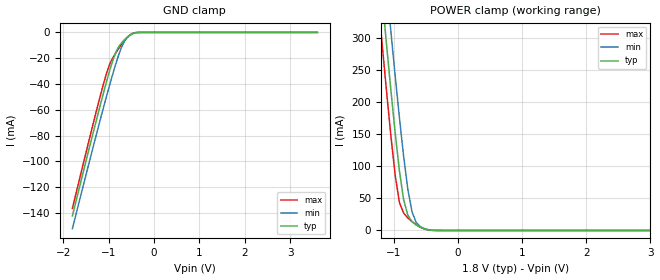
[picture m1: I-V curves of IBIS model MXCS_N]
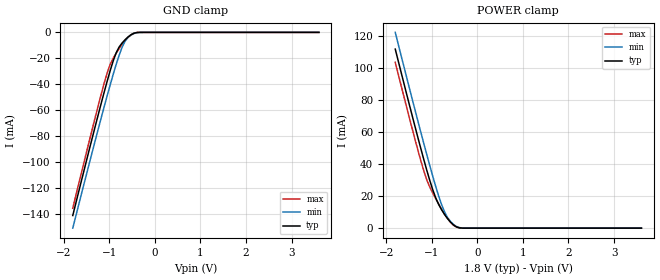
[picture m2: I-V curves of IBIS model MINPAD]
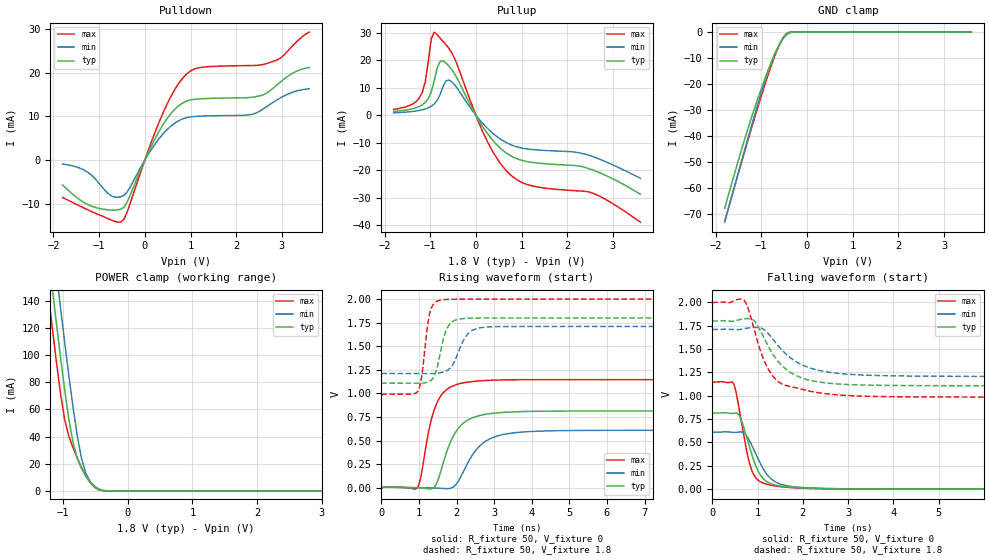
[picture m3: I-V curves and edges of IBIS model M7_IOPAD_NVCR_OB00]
| Created by SiliconSmart  O-2018.09-SP2-3
[IBIS Ver]   4.0
[File Name]   as10204wa_rev1p4.ibs
[File Rev]   1.4
[Date]   Thursday Mar 21 2024
|[Source]   Avalanche Team
|[Notes]   Generated IBIS models from Silicon Smart
|[Rev 1.0]  Initial Release based on extracted netlist
|   Characterization
|[Rev 1.1]  Update Package RLC
|[Rev 1.2]  Recharacterize MIOPAD with Hspice run in high accuracy mode
|[Rev 1.3]  Recharacterize with Hspice to align with datasheet parameter
|[Rev 1.4]  Update the pin to the package pinout assignment
|[Disclaimer]   THE MODEL LIBRARIES ARE PROVIDED AS IS.
|[Copyright]   Copyright 2019, Avalanche Technology., All Rights Reserved
[Component]   AS10xx204_WSON
[Manufacturer] Avalanche Technology
| CONTENT :
| This file contains IBIS MODEL for PSRAM device
| AS1001204 AS1004204 AS1008204 AS1016204
| USAGE :
| The models are derived for the 1.71V to 2.0V I/O Operation.
| Temperatures for model generation: typ: 25, max: -40, min: 105
| Voltages : typ: 1.8V, min: 1.71V, max: 2.0V
| PACKAGES SUPPORTED :
| 8-pad WSON (5.0mm x 6.0mm)
| VERIFICATION :
| Errors  : 0
| Warnings: 30
| All warnings due to non-monotonic data
[Package]
|variable   typ   min   max
R_pkg   8.90E-04   8.89E-04  8.91E-04
L_pkg   1.185E-09  1.18E-09  1.19E-09
C_pkg   2.30E-13   2.21E-13  2.39E-13
[Pin]   signal_name   model_name   R_pin   L_pin   C_pin
1   CS#   MXCS_N   1.05E-01  1.35E-09  9.16E-14
2   SO   MIOPAD   1.05E-01  1.35E-09  9.16E-14
3   WP#   MIOPAD   1.05E-01  1.35E-09  9.16E-14
5   SI   MIOPAD   3.75E-02  3.89E-10  4.24E-14
6   CLK   MINPAD   3.75E-02  3.89E-10  4.24E-14
7   IO_3   MIOPAD   3.75E-02  3.89E-10  4.24E-14
4   VSS   GND   NA   NA   NA
8   VCC   POWER   NA   NA   NA
[Model Selector] MIOPAD
| Model Description
M0_IOPAD_NVCR_OB07   20 Ohms drv strength
M1_IOPAD_NVCR_OB06   30 Ohms drv strength
M2_IOPAD_NVCR_OB05   60 Ohms drv strength
M3_IOPAD_NVCR_OB04   45 Ohms drv strength
M4_IOPAD_NVCR_OB03   70 Ohms drv strength
M5_IOPAD_NVCR_OB02   90 Ohms drv strength
M6_IOPAD_NVCR_OB01   120 Ohms drv strength
M7_IOPAD_NVCR_OB00   45 Ohms drv strength
| Models and submodels in the file (10): MXCS_N (Input), MINPAD (Input), M7_IOPAD_NVCR_OB00 (I/O), M3_IOPAD_NVCR_OB04 (I/O), M5_IOPAD_NVCR_OB02 (I/O), M1_IOPAD_NVCR_OB06 (I/O), M6_IOPAD_NVCR_OB01 (I/O), M2_IOPAD_NVCR_OB05 (I/O), M4_IOPAD_NVCR_OB03 (I/O), M0_IOPAD_NVCR_OB07 (I/O)
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| XCS_N
[Model] MXCS_N
Model_type Input
Enable   Active-High
Vinl  =  0.54
Vinh  =  1.26
| Capacitance  typ   min   max
C_comp   3.084351e-12   2.813138e-12   3.400928e-12
| Variables   typ   min   max
[GND Clamp Reference]   0   0   0
[POWER Clamp Reference]   1.8   1.71   2
[Pulldown Reference]   0   0   0
[Pullup Reference]   1.8   1.71   2
[Temperature Range]   25   105   -40
[Voltage Range]   1.8   1.71   2
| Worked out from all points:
|   GND clamp passes 1 mA (typ) near -0.48 V on its own axis
|   POWER clamp passes 1 mA (typ) near -0.46 V on its own axis
[GND Clamp]
| Voltage   I(typ)   I(min)   I(max)
-1.8V     -142.2mA   -152mA     -136.3mA
-1.303V   -72.38mA   -83.46mA   -65.31mA
-1.173V   -54.66mA   -65.96mA   -47.51mA
-1.043V   -37.59mA   -48.87mA   -31.14mA
-977.6mV  -29.52mA   -40.56mA   -24.56mA
-847.2mV  -15.78mA   -24.8mA    -16.17mA
-716.9mV  -8.18mA    -11.5mA    -9.334mA
-651.7mV  -5.669mA   -6.824mA   -6.326mA
-586.6mV  -3.535mA   -3.869mA   -3.746mA
-456.2mV  -640.4uA   -879uA     -510.8uA
-325.9mV  -14.45uA   -51.53uA   -3.775uA
3.6V      0A         0A         0A
[POWER Clamp]
| Voltage   I(typ)   I(min)   I(max)
-1.8V     1.062A     1.152A     991.6mA
-1.238V   424.5mA    517.2mA    351.4mA
-1.173V   353.2mA    445.8mA    280.1mA
-1.108V   283.2mA    375.4mA    210.6mA
-1.043V   215.2mA    306.4mA    144.3mA
-977.6mV  150.6mA    239.2mA    85.02mA
-912.4mV  92.52mA    174.9mA    43.53mA
-847.2mV  47.97mA    115.2mA    27.04mA
-716.9mV  13.61mA    29.16mA    13.92mA
-651.7mV  8.604mA    12.47mA    8.943mA
-325.9mV  22.75uA    80.1uA     9.962uA
3.6V      0A         0A         0A
| INPAD
[Model] MINPAD
Model_type Input
Enable   Active-High
Vinl  =  0.54
Vinh  =  1.26
| Capacitance  typ   min   max
C_comp   2.700843e-12   2.498345e-12   2.928788e-12
| Variables   typ   min   max
[GND Clamp Reference]   0   0   0
[POWER Clamp Reference]   1.8   1.71   2
[Pulldown Reference]   0   0   0
[Pullup Reference]   1.8   1.71   2
[Temperature Range]   25   105   -40
[Voltage Range]   1.8   1.71   2
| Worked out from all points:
|   GND clamp passes 1 mA (typ) near -0.48 V on its own axis
|   POWER clamp passes 1 mA (typ) near -0.47 V on its own axis
[GND Clamp]
| Voltage   I(typ)   I(min)   I(max)
-1.8V     -141.2mA   -150.9mA   -135.5mA
-1.303V   -71.9mA    -82.87mA   -64.94mA
-1.173V   -54.3mA    -65.5mA    -47.25mA
-1.043V   -37.35mA   -48.53mA   -30.99mA
-977.6mV  -29.34mA   -40.29mA   -24.44mA
-847.2mV  -15.7mA    -24.65mA   -16.09mA
-716.9mV  -8.148mA   -11.44mA   -9.29mA
-651.7mV  -5.65mA    -6.8mA     -6.299mA
-586.6mV  -3.525mA   -3.859mA   -3.733mA
-456.2mV  -639.6uA   -877.8uA   -510.2uA
-325.9mV  -14.45uA   -51.53uA   -3.775uA
3.6V      0A         0A         0A
[POWER Clamp]
| Voltage   I(typ)   I(min)   I(max)
-1.8V     111.7mA    122.1mA    103.4mA
-1.369V   63.57mA    73.93mA    55.54mA
-1.238V   49.53mA    59.72mA    41.97mA
-1.108V   36.07mA    45.8mA     30.06mA
-977.6mV  23.92mA    32.38mA    21.88mA
-912.4mV  18.87mA    26mA       18.39mA
-782.1mV  11.36mA    14.53mA    11.73mA
-651.7mV  5.917mA    6.557mA    5.926mA
-521.4mV  1.955mA    2.241mA    1.736mA
-391mV    174.8uA    333.4uA    115.2uA
-260.7mV  2.189uA    12.94uA    482.3nA
3.6V      0A         0A         0A
[Model] M7_IOPAD_NVCR_OB00
Model_type I/O
Enable   Active-High
Vinl  =  0.54
Vinh  =  1.26
Vmeas =  0.9
Cref  =  30e-12
| Capacitance  typ   min   max
C_comp   3.869840e-12   3.575244e-12   4.208825e-12
| Variables   typ   min   max
[GND Clamp Reference]   0   0   0
[POWER Clamp Reference]   1.8   1.71   2
[Pulldown Reference]   0   0   0
[Pullup Reference]   1.8   1.71   2
[Temperature Range]   25   105   -40
[Voltage Range]   1.8   1.71   2
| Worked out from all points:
|   slope of the pulldown table from 0 to 0.27 V, typ, clamps not added: 46.6 ohm
|   slope of the pullup table from 0 to 0.27 V, typ, clamps not added: 38.6 ohm
|   GND clamp passes 1 mA (typ) near -0.46 V on its own axis
|   POWER clamp passes 1 mA (typ) near -0.44 V on its own axis
|   falling waveform, R_fixture 50, V_fixture 0: 20-80 % time 347ps typ, 419ps min, 280ps max; typ from 0.814 V to 0 V
|   falling waveform, R_fixture 50, V_fixture 1.8: 20-80 % time 649ps typ, 769ps min, 500ps max; typ from 1.8 V to 1.1 V
|   rising waveform, R_fixture 50, V_fixture 0: 20-80 % time 520ps typ, 636ps min, 397ps max; typ from 0 V to 0.814 V
|   rising waveform, R_fixture 50, V_fixture 1.8: 20-80 % time 256ps typ, 352ps min, 184ps max; typ from 1.1 V to 1.8 V
[GND Clamp]
| Voltage   I(typ)   I(min)   I(max)
-1.8V     -67.84mA   -73.19mA   -72.81mA
-1.499V   -49.26mA   -53.93mA   -54.28mA
-1.303V   -37.87mA   -41.64mA   -42.4mA
-1.108V   -27.29mA   -29.68mA   -30.84mA
-912.4mV  -17.6mA    -18.46mA   -19.84mA
-782.1mV  -11.7mA    -11.87mA   -13.01mA
-651.7mV  -6.447mA   -6.494mA   -6.896mA
-521.4mV  -2.255mA   -2.526mA   -2.141mA
-456.2mV  -849.3uA   -1.156mA   -679.4uA
-391mV    -172uA     -356.5uA   -88.88uA
-260.7mV  -2.088uA   -12.98uA   -254.3nA
3.6V      0A         0A         0A
[POWER Clamp]
| Voltage   I(typ)   I(min)   I(max)
-1.8V     419.8mA    456.6mA    390.9mA
-1.238V   178mA      215.7mA    148.4mA
-1.173V   151mA      188.6mA    121.7mA
-1.108V   124.5mA    161.8mA    96mA
-1.043V   98.85mA    135.4mA    72.14mA
-977.6mV  74.56mA    109.6mA    52.56mA
-912.4mV  52.76mA    84.78mA    40.16mA
-847.2mV  35.48mA    61.36mA    31.71mA
-716.9mV  16.42mA    23.91mA    17.31mA
-651.7mV  10.9mA     13.27mA    11.28mA
-456.2mV  1.168mA    1.554mA    921.1uA
3.6V      0A         0A         0A
[Pulldown]
| Voltage   I(typ)   I(min)   I(max)
-1.8V     -5.69mA    -910.5uA   -8.548mA
-1.173V   -10.5mA    -3.41mA    -11.73mA
-782.1mV  -11.39mA   -7.821mA   -13.47mA
-521.4mV  -11.21mA   -8.363mA   -14.11mA
-391mV    -9.672mA   -7.354mA   -11.98mA
372.4mV   7.658mA    5.676mA    10.17mA
869mV     13.26mA    9.551mA    19.2mA
1.241V    14.01mA    10.05mA    21.19mA
2.352V    14.36mA    10.46mA    21.6mA
2.766V    16.04mA    12.9mA     22.39mA
3.248V    19.92mA    15.56mA    26.27mA
3.6V      21.15mA    16.29mA    29.24mA
[Pullup]
| Voltage   I(typ)   I(min)   I(max)
-1.8V     1.352mA    850uA      2.099mA
-1.238V   3.177mA    1.737mA    6.26mA
-1.108V   4.622mA    2.263mA    12.15mA
-977.6mV  8.411mA    3.225mA    27.68mA
-912.4mV  12.48mA    4.062mA    30.16mA
-782.1mV  19.57mA    7.55mA     27.92mA
-586.6mV  17.73mA    12.75mA    24.14mA
248.3mV   -6.519mA   -4.68mA    -9.425mA
744.8mV   -14.56mA   -10.55mA   -21.44mA
1.241V    -17.12mA   -12.46mA   -25.69mA
2.559V    -19.89mA   -15mA      -28.27mA
3.6V      -28.69mA   -22.89mA   -38.81mA
[Ramp]
dV/dt_r   0.488568/0.519945n  0.365787/0.635811n  0.687926/0.397312n
dV/dt_f   0.417076/0.649039n  0.300973/0.768787n  0.608145/0.500349n
R_load = 50
[Falling Waveform]
R_fixture = 50
V_fixture = 0
V_fixture_min = 0
V_fixture_max = 0
| Time   V(typ)   V(min)   V(max)
0s        814.3mV    609.6mV    1.147V
474ps     813.8mV    607.7mV    1.125V
599.7ps   783.2mV    612.6mV    837.3mV
776.9ps   525.9mV    556.8mV    365.8mV
948.2ps   264.1mV    391.6mV    129.1mV
1.058ns   153.3mV    278.2mV    80.21mV
1.23ns    73.11mV    143.7mV    48.66mV
1.546ns   30.54mV    48.34mV    24.51mV
3.663ns   898uV      1.414mV    777.2uV
21.88ns   242.1nV    617.1nV    249.8nV
[Falling Waveform]
R_fixture = 50
V_fixture = 1.8
V_fixture_min = 1.71
V_fixture_max = 2
| Time   V(typ)   V(min)   V(max)
0s        1.8V       1.71V      2V
684.9ps   1.824V     1.718V     2.031V
791.9ps   1.828V     1.727V     1.935V
954.3ps   1.787V     1.732V     1.656V
1.128ns   1.633V     1.714V     1.397V
1.355ns   1.433V     1.596V     1.2V
1.831ns   1.222V     1.372V     1.089V
2.549ns   1.136V     1.255V     1.02V
4.579ns   1.109V     1.211V     987.9mV
21.88ns   1.105V     1.208V     986.4mV
[Rising Waveform]
R_fixture = 50
V_fixture = 0
V_fixture_min = 0
V_fixture_max = 0
| Time   V(typ)   V(min)   V(max)
0s        74.44nV    376.1nV    131.9nV
944.2ps   468.1uV    1.945mV    -6.144mV
1.049ns   -1.961mV   1.585mV    113mV
1.314ns   -12.28mV   -657.4uV   697.4mV
1.509ns   84.57mV    -3.643mV   925.6mV
1.949ns   574.2mV    19.61mV    1.087V
2.418ns   740.7mV    345.5mV    1.126V
3.037ns   792.2mV    543.4mV    1.141V
4.152ns   810.9mV    599.7mV    1.146V
21.88ns   814.3mV    609.6mV    1.147V
[Rising Waveform]
R_fixture = 50
V_fixture = 1.8
V_fixture_min = 1.71
V_fixture_max = 2
| Time   V(typ)   V(min)   V(max)
0s        1.105V     1.208V     986.4mV
973.3ps   1.108V     1.21V      1.024V
1.065ns   1.109V     1.21V      1.158V
1.296ns   1.131V     1.21V      1.861V
1.443ns   1.219V     1.212V     1.968V
1.614ns   1.514V     1.223V     1.992V
1.902ns   1.764V     1.306V     1.998V
2.276ns   1.796V     1.619V     1.999V
2.814ns   1.799V     1.704V     1.999V
21.88ns   1.8V       1.71V      2V
